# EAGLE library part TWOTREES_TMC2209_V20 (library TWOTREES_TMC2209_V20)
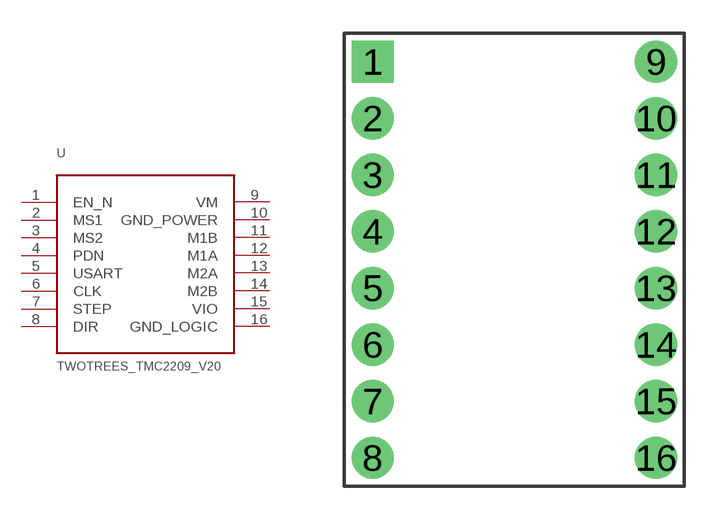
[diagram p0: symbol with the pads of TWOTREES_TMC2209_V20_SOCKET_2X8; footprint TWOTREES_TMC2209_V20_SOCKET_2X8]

Designator prefix U

## TWOTREES_TMC2209_V20  [TWOTREES_TMC2209_V20_SOCKET_2X8]
1  EN_N  in
2  MS1  in
3  MS2  in
4  PDN  pas
5  USART  pas
6  CLK  pas
7  STEP  in
8  DIR  in
9  VM  pwr
10  GND_POWER  pas
11  M1B  out
12  M1A  out
13  M2A  out
14  M2B  out
15  VIO  pwr
16  GND_LOGIC  pas

## Footprint TWOTREES_TMC2209_V20_SOCKET_2X8 (pad centres in mm)
drill 1 pad 1.9 square: 1 -6.35,8.89
drill 1 pad 1.9 round: 2 -6.35,6.35; 3 -6.35,3.81; 4 -6.35,1.27; 5 -6.35,-1.27; 6 -6.35,-3.81; 7 -6.35,-6.35; 8 -6.35,-8.89; 9 6.35,8.89; 10 6.35,6.35; 11 6.35,3.81; 12 6.35,1.27; 13 6.35,-1.27; 14 6.35,-3.81; 15 6.35,-6.35; 16 6.35,-8.89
